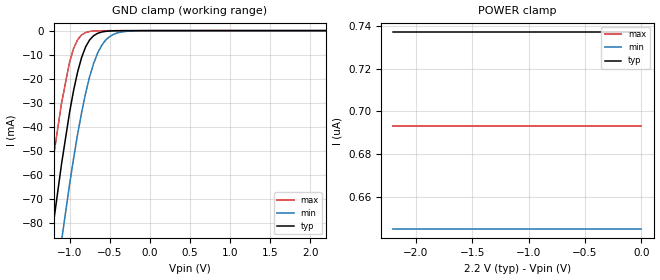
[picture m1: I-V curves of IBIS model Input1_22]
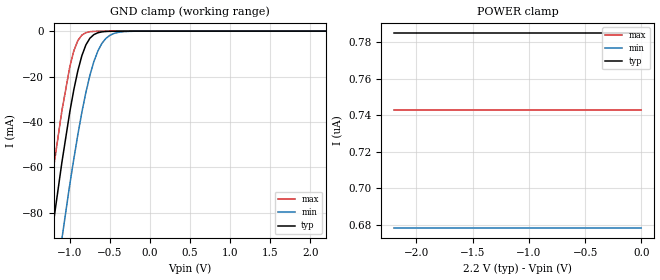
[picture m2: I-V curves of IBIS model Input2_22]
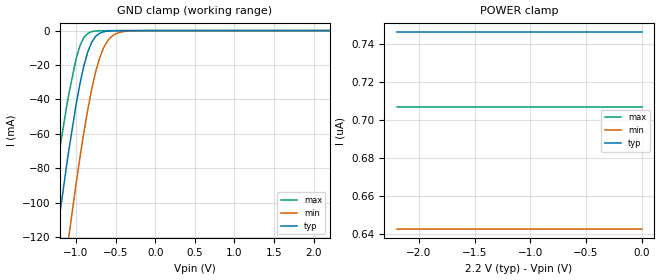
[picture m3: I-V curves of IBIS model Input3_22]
|//////////////////////////////////////////////////////////////////////////////
|//////////////////////////////////////////////////////////////////////////////
|   @@@@@@@   @@@@@@@   @@@@@@@   @@@@@@@   @@@@@@@   @@@@@@   @@
|   @@@@@@@@@   @@@@@@@@@   @@@@@@@@@   @@@@@@@@@   @@@@@@@@@ @@@@@@@@  @
|   @@@   @@@ @@@   @@@ @@@   @@@   @@@ @@@   @@@@   @@@  @
|   @@   @@ @@   @@ @@@@@@@@@@@ @@@@@@@@@@@ @@   @@   @@ @@
|   @@@   @@@ @@   @@   @@@ @@@   @@   @@   @@ @@
|   @@@@@@@@@  @@   @@  @@@@@@@@@   @@@@@@@@@  @@   @@   @@ @@
|   @@@@@@@   @@   @@   @@@@@@@   @@@@@@@   @@   @@   @@ @@
|   IBIS Model of CAV24C32
|   EEPROM Serial 32-Kb I2C Automotive Grade 1
|   WLCSP-4 Package Type, CASE 567JY, C4C SUFFIX
|   SOIC-8  Package Type, CASE 751BD,   W SUFFIX
|   TSSOP-8 Package Type, CASE 948AL,   Y SUFFIX
|   The model is covering the following Vccs:
|   2.2V, 3.3V, 5.0V
|//////////////////////////////////////////////////////////////////////////////
|//////////////////////////////////////////////////////////////////////////////
[IBIS Ver]   3.2
|   7.2 compatible
|//////////////////////////////////////////////////////////////////////////////
[Comment Char] |_char
|//////////////////////////////////////////////////////////////////////////////
[File Name]   cav24c32_ga_r0.ibs
|//////////////////////////////////////////////////////////////////////////////
[File Rev]   0.0
|   0.0 - Sep 20, 2024 - File created
|//////////////////////////////////////////////////////////////////////////////
[Date]   September 20, 2024
|//////////////////////////////////////////////////////////////////////////////
[Source]   Measurements and simulations at onsemi
|//////////////////////////////////////////////////////////////////////////////
[Notes]
   - The currents greater than +/- 100 mA are extrapolated
   - The non-monotonic behavior of GND Clamp and Pulldown
   curves are expected
|//////////////////////////////////////////////////////////////////////////////
[Disclaimer]
   - onsemi Corporation hereby grants
   the user of this IBIS model a license to use this IBIS
   model under the following terms. This license in nonexclusive
   and nontransferable. Before using this IBIS model.
   After reading the terms and conditions of this license,
   the user either must accept these terms,
   or the IBIS model should be returned to onsemi within 30 days.
   - The user is hereby granted a license to use the IBIS model.
   This shall not be construed as a right to sell,
   or otherwise profit either by leasing or renting this software.
   - The user may modify the IBIS model to suit his specific
   applications but rights to derivative works and such
   modifications shall belong to onsemi.
   - This IBIS model is provided on an "as is" basis.
   onsemi makes absolutely no warranty with respect
   to the information contained herein.
   By use of this IBIS model, the user assumes full risk as to the
   quality and suitablility of the model to his particular use,
   and by using this model assumes the entire risk.
   Under all circumstances the user shall not hold
   onsemi liable in any way for the results obtained.
   onsemi reserves the right to make to improve
   the model for reliability, function, or design.
   onsemi does not convey any license under patent
   rights or any other intellectual property rights,
   including those of third parties.
   - onsemi is not obligated to provide maintenance
   or support for the licensed IBIS model.
   - Cont onsemi at ATTN:LOGIC APPLICATIONS/IBIS MODEL.
   5701 N Pima Rd, Scottsdale, AZ 85250
|//////////////////////////////////////////////////////////////////////////////
[Copyright]   (c) 2024 onsemi Corp.
|//////////////////////////////////////////////////////////////////////////////
|//////////////////////////////////////////////////////////////////////////////
[Component]   CAV24C32C4CTR
|//////////////////////////////////////////////////////////////////////////////
[Manufacturer]  onsemi
|   Data Sheet: CAV24C32/D, Rev. 6,  Aug, 2024
|//////////////////////////////////////////////////////////////////////////////
[Package]
|  WLCSP-4
| C4C SUFFIX
| CASE 567JY
| variable   typ   min   max
R_pkg   0.0059   0.0053   0.0065
L_pkg   0.2525nH   0.2200nH   0.2700nH
C_pkg   0.6275pF   0.6000pF   0.6600pF
|//////////////////////////////////////////////////////////////////////////////
[Pin]   signal_name   model_name   R_pin   L_pin   C_pin
A1   VCC   POWER   0.0065   0.2600nH   0.6000pF
A2   VSS   GND   0.0063   0.2200nH   0.6600pF
B1   SCL   Input4   0.0054   0.2600nH   0.6400pF
B2   SDA   I/O   0.0053   0.2700nH   0.6100pF
|//////////////////////////////////////////////////////////////////////////////
[Component]   CAV24C32WE-GT3
|//////////////////////////////////////////////////////////////////////////////
[Manufacturer]  onsemi
|   Data Sheet: CAV24C32/D, Rev. 6,  Aug, 2024
|//////////////////////////////////////////////////////////////////////////////
[Package]
|   SOIC-8
| CASE 751BD
|  W SUFFIX
| variable   typ   min   max
R_pkg   0.0256   0.0171   0.0370
L_pkg   2.5734nH   2.1811nH   3.0947nH
C_pkg   0.2631pF   0.2247pF   0.3139pF
|//////////////////////////////////////////////////////////////////////////////
[Pin]   signal_name   model_name   R_pin   L_pin   C_pin
1   A0   Input1   0.0256   2.5734nH   0.2631pF
2   A1   Input2   0.0171   2.1830nH   0.2255pF
3   A2   Input3   0.0187   2.1813nH   0.2247pF
4   GND   GND   0.0350   3.0935nH   0.3131pF
5   SDA   I/O   0.0357   3.0942nH   0.3139pF
6   SCL   Input4   0.0172   2.1860nH   0.2251pF
7   WP   Input5   0.0187   2.1811nH   0.2257pF
8   VCC   POWER   0.0370   3.0947nH   0.3137pF
|//////////////////////////////////////////////////////////////////////////////
[Component]   CAV24C32YE-GT3
|//////////////////////////////////////////////////////////////////////////////
[Manufacturer]  onsemi
|   Data Sheet: CAV24C32/D, Rev. 6,  Aug, 2024
|//////////////////////////////////////////////////////////////////////////////
[Package]
|   TSSOP-8
| CASE 948AL
|  Y SUFFIX
| variable   typ   min   max
R_pkg   0.0402   0.0348   0.0463
L_pkg   2.5922nH   2.4111nH   2.8670nH
C_pkg   0.3019pF   0.286pF   0.3226pF
|//////////////////////////////////////////////////////////////////////////////
[Pin]   signal_name   model_name   R_pin   L_pin   C_pin
1   A0   Input1   0.0402   2.5922nH   0.3019pF
2   A1   Input2   0.0376   2.4380nH   0.2860pF
3   A2   Input3   0.0348   2.4111nH   0.2871pF
4   GND   GND   0.0435   2.7843nH   0.3226pF
5   SDA   I/O   0.0448   2.7854nH   0.3210pF
6   SCL   Input5   0.0364   2.4210nH   0.2875pF
7   WP   Input5   0.0381   2.4386nH   0.2871pF
8   VCC   POWER   0.0463   2.8670nH   0.3223pF
|//////////////////////////////////////////////////////////////////////////////
|//////////////////////////////////////////////////////////////////////////////
[Model Selector]   Input1
Input1_22   Vcc = 2.20
Input1_33   Vcc = 3.30
Input1_50   Vcc = 5.00
|//////////////////////////////////////////////////////////////////////////////
[Model Selector]   Input2
Input2_22   Vcc = 2.20
Input2_33   Vcc = 3.30
Input2_50   Vcc = 5.00
|//////////////////////////////////////////////////////////////////////////////
[Model Selector]   Input3
Input3_22   Vcc = 2.20
Input3_33   Vcc = 3.30
Input3_50   Vcc = 5.00
|//////////////////////////////////////////////////////////////////////////////
[Model Selector]   Input4
Input4_22   Vcc = 2.20
Input4_33   Vcc = 3.30
Input4_50   Vcc = 5.00
|//////////////////////////////////////////////////////////////////////////////
[Model Selector]   Input5
Input5_22   Vcc = 2.20
Input5_33   Vcc = 3.30
Input5_50   Vcc = 5.00
|//////////////////////////////////////////////////////////////////////////////
[Model Selector]   I/O
I/O_22   Vcc = 2.20
I/O_33   Vcc = 3.30
I/O_50   Vcc = 5.00
| Models and submodels in the file (18): Input1_22 (Input), Input2_22 (Input), Input3_22 (Input), Input4_22 (Input), Input5_22 (Input), I/O_22 (I/O_open_drain), Input1_33 (Input), Input2_33 (Input), Input3_33 (Input), Input4_33 (Input), Input5_33 (Input), I/O_33 (I/O_open_drain), Input1_50 (Input), Input2_50 (Input), Input3_50 (Input), Input4_50 (Input), Input5_50 (Input), I/O_50 (I/O_open_drain)
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|//////////////////////////////////////////////////////////////////////////////
|//////////////////////////////////////////////////////////////////////////////
[Model]  Input1_22
Model_type Input
Vinh =  1.54
Vinl =  0.66
|  variable   typ   min   max
C_comp   6pF   NA   6pF
|//////////////////////////////////////////////////////////////////////////////
[Temperature Range]   25   NA   -40
|//////////////////////////////////////////////////////////////////////////////
[Voltage Range]   2.20V   NA   2.70V
|//////////////////////////////////////////////////////////////////////////////
[POWER Clamp Reference] 2.20V   NA   2.70V
|//////////////////////////////////////////////////////////////////////////////
[GND Clamp Reference]   0V   NA   0V
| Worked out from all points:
|   GND clamp passes 1 mA (typ) near -0.64 V on its own axis
|//////////////////////////////////////////////////////////////////////////////
[GND Clamp]
|   Voltage   I(typ)   I(min)   I(max)
-2.2V     -375mA     -408mA     -342mA
-1.4V     -134mA     -167mA     -104mA
-1.3V     -106mA     -140mA     -77.5mA
-1.2V     -79.8mA    -113mA     -52.3mA
-1.1V     -55.4mA    -87.4mA    -30.1mA
-1V       -34mA      -63.9mA    -13.1mA
-950mV    -24.9mA    -53.2mA    -7.42mA
-800mV    -6.76mA    -26mA      -791uA
-700mV    -2.1mA     -13.6mA    -158uA
-600mV    -578uA     -6.14mA    -40.4uA
-400mV    -45.5uA    -921uA     -11.2uA
2.2V      737nA      645nA      693nA
|//////////////////////////////////////////////////////////////////////////////
[POWER Clamp]
|   Voltage   I(typ)   I(min)   I(max)
-2.2V     737nA      645nA      693nA
-2.1V     737nA      645nA      693nA
-2V       737nA      645nA      693nA
0V        737nA      645nA      693nA
|//////////////////////////////////////////////////////////////////////////////
|//////////////////////////////////////////////////////////////////////////////
[Model]  Input2_22
Model_type Input
Vinh =  1.54
Vinl =  0.66
|  variable   typ   min   max
C_comp   6pF   NA   6pF
|//////////////////////////////////////////////////////////////////////////////
[Temperature Range]   25   NA   -40
|//////////////////////////////////////////////////////////////////////////////
[Voltage Range]   2.20V   NA   2.70V
|//////////////////////////////////////////////////////////////////////////////
[POWER Clamp Reference] 2.20V   NA   2.70V
|//////////////////////////////////////////////////////////////////////////////
[GND Clamp Reference]   0V   NA   0V
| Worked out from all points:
|   GND clamp passes 1 mA (typ) near -0.67 V on its own axis
|//////////////////////////////////////////////////////////////////////////////
[GND Clamp]
|   Voltage   I(typ)   I(min)   I(max)
-2.2V     -376mA     -407mA     -354mA
-1.3V     -110mA     -144mA     -85.8mA
-1.2V     -83mA      -117mA     -59.3mA
-1.1V     -57.9mA    -91.5mA    -35.2mA
-1V       -35.4mA    -67.3mA    -15.6mA
-950mV    -25.7mA    -56.1mA    -8.65mA
-900mV    -17.4mA    -45.5mA    -4.12mA
-800mV    -6.06mA    -27mA      -664uA
-700mV    -1.52mA    -13.4mA    -103uA
-600mV    -328uA     -5.39mA    -26.6uA
-400mV    -21.2uA    -570uA     -10.6uA
2.2V      785nA      678nA      743nA
|//////////////////////////////////////////////////////////////////////////////
[POWER Clamp]
|   Voltage   I(typ)   I(min)   I(max)
-2.2V     785nA      678nA      743nA
-2.1V     785nA      678nA      743nA
-2V       785nA      678nA      743nA
0V        785nA      678nA      743nA
|//////////////////////////////////////////////////////////////////////////////
|//////////////////////////////////////////////////////////////////////////////
[Model]  Input3_22
Model_type Input
Vinh =  1.54
Vinl =  0.66
|  variable   typ   min   max
C_comp   6pF   NA   6pF
|//////////////////////////////////////////////////////////////////////////////
[Temperature Range]   25   NA   -40
|//////////////////////////////////////////////////////////////////////////////
[Voltage Range]   2.20V   NA   2.70V
|//////////////////////////////////////////////////////////////////////////////
[POWER Clamp Reference] 2.20V   NA   2.70V
|//////////////////////////////////////////////////////////////////////////////
[GND Clamp Reference]   0V   NA   0V
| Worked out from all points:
|   GND clamp passes 1 mA (typ) near -0.67 V on its own axis
|//////////////////////////////////////////////////////////////////////////////
[GND Clamp]
|   Voltage   I(typ)   I(min)   I(max)
-2.2V     -484mA     -568mA     -412mA
-1.4V     -175mA     -236mA     -131mA
-1.3V     -139mA     -197mA     -98.2mA
-1.2V     -105mA     -159mA     -67.2mA
-1.1V     -72.3mA    -123mA     -39.1mA
-1V       -43.3mA    -89.3mA    -16.5mA
-950mV    -30.9mA    -73.6mA    -8.79mA
-850mV    -12.2mA    -45.5mA    -1.56mA
-750mV    -3.25mA    -23.6mA    -213uA
-650mV    -680uA     -9.8mA     -40.1uA
-450mV    -32.3uA    -1.01mA    -12.2uA
2.2V      746nA      643nA      707nA
|//////////////////////////////////////////////////////////////////////////////
[POWER Clamp]
|   Voltage   I(typ)   I(min)   I(max)
-2.2V     746nA      643nA      707nA
-2.1V     746nA      643nA      707nA
-2V       746nA      643nA      707nA
0V        746nA      643nA      707nA
